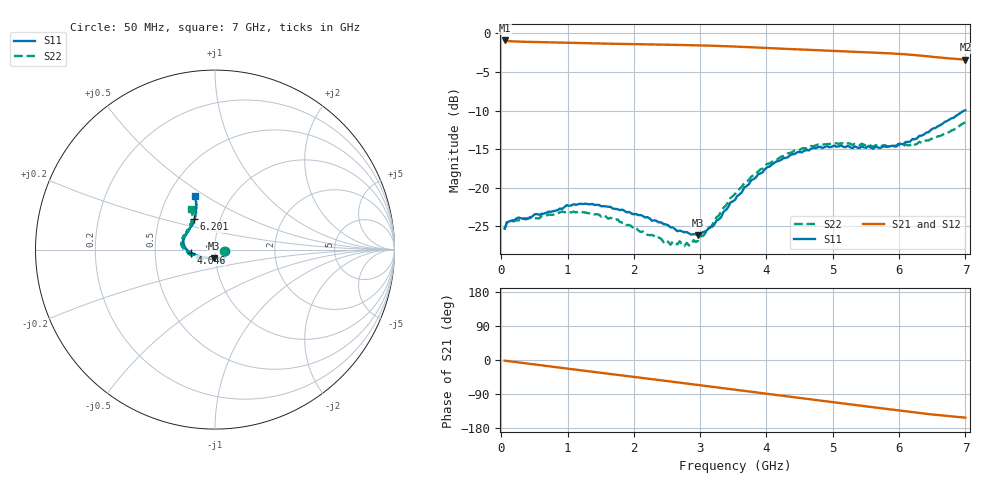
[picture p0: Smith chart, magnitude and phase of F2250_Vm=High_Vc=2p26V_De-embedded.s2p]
! Integrated Device Technology
! Corporate Headquarters
! 6024 Silver Creek Valley Road
! San Jose, CA 95138  USA
! Phone:  1-408-284-8200
! Toll Free:  1-800-223-1366
! Webpage:  http://www.idt.com/
! Timing and RF Division
! 515 Groton Road, Suite 102
! Westford, MA 01886-6024
! Device:  F2250
! Description: Voltage Variable RF Attenuator
! Frequency:  50.0 -  6000.00 MHz
! Package:  3x3 mm Thin QFN Plastic Package: 16 pin
! Ports:  2 RF, 3 DC
!  Pin  1  = GND
!  Pin  2  = NC
!  Pin  3  = RF1  = Port 1
!  Pin  4  = NC
!  Pin  5  = GND
!  Pin  6  = GND
!  Pin  7  = GND
!  Pin  8  = GND
!  Pin  9  = NC
!  Pin 10  = RF2  = Port 2
!  Pin 11  = NC
!  Pin 12  = GND
!  Pin 13  = GND
!  Pin 14  = VCNTRL
!  Pin 15  = VDD
!  Pin 16  = VMODE
! Vcntrl:  2.260 Volts
! Vmode:  +3.300 Volts
! Vdd:  +3.30  Volts
! Current:  1.315 mA
! Data:  The device was measured on a the F2250 evaluation board which has
!  individual transmission lines to the RF pins.  Data was collected
!  using a calibrated network analyzer.  The evaluation board was
!  de-embedded using a TRL calibration technique.
!  The reference plane is the edge of the package pin.
! Misc:  SN 10
!  Action Tracker AT0258
! Date Measured:  2014-11-26
! Date:  2015-10-15  MJV
! Note:
!  Integrated Device Technology supplies this data as a sample of measured
!  data at the package pin for this product.  Your particular data for this
!  product may vary.
!  Data was taken at 25 degrees C.
!  Integrated Device Technology reserves the right to change this data at anytime.
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# GHz S dB R 50
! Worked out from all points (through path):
!   201 points, 50 MHz to 7 GHz, reference 50 ohm
!   highest |S21| = -0.91 dB at 50 MHz (marker M1); lowest = -3.4 dB at 7 GHz (marker M2)
!   group delay of S21, straight-line fit = 61.1 ps
!   lowest |S11| = -26.2 dB at 2.969 GHz (marker M3), VSWR 1.10, Z = 49.3 - j4.83 ohm
!   |S11| at or under -10 dB: start of sweep to 6.988 GHz
!   |S22| runs from -27.6 to -11.5 dB; largest |S21 - S12| = 0.0019
!   S11 on the Smith chart (normalised r, x): 50 MHz: 1.11, -0.02; 4.046 GHz: 0.76, -0.03; 6.201 GHz: 0.75, +0.27; 7 GHz: 0.68, +0.45
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0.05  -25.26 -10.2  -0.91 -1.8  -0.91 -1.8  -25.43 -10.5
0.1195  -24.36 -9.9  -1.01 -3.2  -1.01 -3.2  -24.32 -8.7
0.91875  -22.73 -48.9  -1.20 -21.0  -1.20 -21.1  -23.05 -50.3
1.2315  -22.11 -56.6  -1.26 -27.9  -1.26 -27.9  -23.17 -60.8
1.75275  -22.77 -63.6  -1.36 -39.1  -1.35 -39.1  -24.07 -67.4
2.37825  -24.49 -63.4  -1.45 -52.8  -1.45 -52.8  -26.44 -67.5
2.552  -25.12 -68.1  -1.47 -56.7  -1.47 -56.7  -27.38 -73.9
2.691  -25.55 -75.9  -1.50 -59.8  -1.50 -59.8  -26.92 -81.4
2.7605  -25.77 -78.0  -1.51 -61.3  -1.51 -61.3  -27.56 -85.8
2.969  -26.18 -95.4  -1.55 -66.0  -1.55 -66.0  -26.85 -104.8
3.21225  -24.78 -125.5  -1.61 -71.5  -1.61 -71.5  -24.21 -129.7
3.4555  -21.91 -146.6  -1.68 -77.0  -1.68 -77.0  -21.33 -145.0
3.525  -21.57 -151.0  -1.70 -78.5  -1.70 -78.6  -20.81 -148.2
3.76825  -19.03 -163.5  -1.80 -84.0  -1.80 -84.0  -18.58 -159.2
4.04625  -17.24 -173.0  -1.91 -90.2  -1.91 -90.2  -16.85 -169.7
4.4285  -15.60 176.8  -2.05 -98.6  -2.06 -98.6  -15.13 178.9
4.7065  -14.83 169.8  -2.15 -104.8  -2.16 -104.8  -14.63 173.2
5.054  -14.67 161.6  -2.28 -112.5  -2.28 -112.5  -14.23 166.1
5.85325  -14.65 135.7  -2.58 -130.0  -2.58 -130.1  -14.63 147.3
6.20075  -13.70 124.0  -2.79 -137.7  -2.79 -137.8  -14.22 138.3
6.54825  -12.26 116.0  -3.06 -144.7  -3.06 -144.8  -13.56 127.0
7  -9.97 111.1  -3.39 -152.1  -3.40 -152.2  -11.53 120.7
